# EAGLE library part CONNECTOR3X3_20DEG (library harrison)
3x3 connector, 20 degrees
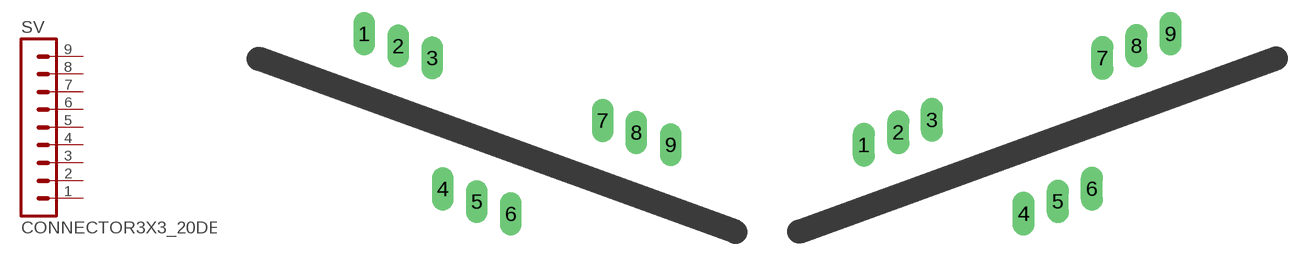
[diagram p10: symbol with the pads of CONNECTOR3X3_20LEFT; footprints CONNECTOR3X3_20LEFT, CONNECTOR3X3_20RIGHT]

Designator prefix SV

## CONNECTOR3X3_20DEG  [CONNECTOR3X3_20LEFT]
1  1  pas
2  2  pas
3  3  pas
4  4  pas
5  5  pas
6  6  pas
7  7  pas
8  8  pas
9  9  pas

## CONNECTOR3X3_20DEGRIGHT  [CONNECTOR3X3_20RIGHT]
Pads as for CONNECTOR3X3_20LEFT

## CONNECTOR3X3_20DEGLEFT  [CONNECTOR3X3_20LEFT]
Pads as for CONNECTOR3X3_20LEFT

## Footprint CONNECTOR3X3_20LEFT (pad centres in mm)
drill 1.016 long: 1 -26.035,13.919; 2 -23.647,13.056; 3 -21.26,12.217; 4 -20.523,3.023; 5 -18.136,2.134; 6 -15.748,1.27; 7 -9.322,7.823; 8 -6.96,6.985; 9 -4.547,6.121

## Footprint CONNECTOR3X3_20RIGHT (pad centres in mm)
drill 1.016 long: 1 4.547,6.096; 2 6.96,6.985; 3 9.322,7.849; 4 15.748,1.27; 5 18.136,2.134; 6 20.523,3.023; 7 21.26,12.192; 8 23.647,13.056; 9 26.035,13.894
